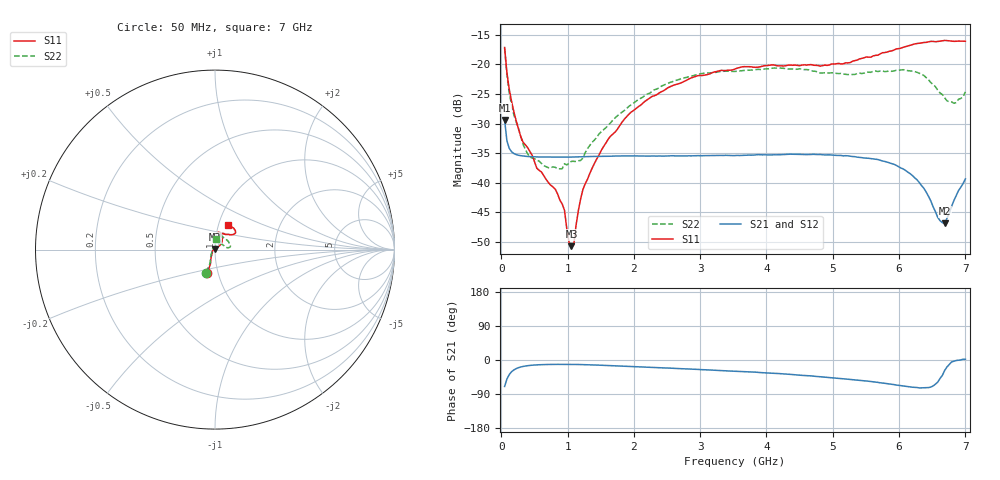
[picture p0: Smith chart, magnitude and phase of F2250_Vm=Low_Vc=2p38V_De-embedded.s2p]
! Integrated Device Technology
! Corporate Headquarters
! 6024 Silver Creek Valley Road
! San Jose, CA 95138  USA
! Phone:  1-408-284-8200
! Toll Free:  1-800-223-1366
! Webpage:  http://www.idt.com/
! Timing and RF Division
! 515 Groton Road, Suite 102
! Westford, MA 01886-6024
! Device:  F2250
! Description: Voltage Variable RF Attenuator
! Frequency:  50.0 -  6000.00 MHz
! Package:  3x3 mm Thin QFN Plastic Package: 16 pin
! Ports:  2 RF, 3 DC
!  Pin  1  = GND
!  Pin  2  = NC
!  Pin  3  = RF1  = Port 1
!  Pin  4  = NC
!  Pin  5  = GND
!  Pin  6  = GND
!  Pin  7  = GND
!  Pin  8  = GND
!  Pin  9  = NC
!  Pin 10  = RF2  = Port 2
!  Pin 11  = NC
!  Pin 12  = GND
!  Pin 13  = GND
!  Pin 14  = VCNTRL
!  Pin 15  = VDD
!  Pin 16  = VMODE
! Vcntrl:  2.380 Volts
! Vmode:  +0.000 Volts
! Vdd:  +3.30  Volts
! Current:  1.177 mA
! Data:  The device was measured on a the F2250 evaluation board which has
!  individual transmission lines to the RF pins.  Data was collected
!  using a calibrated network analyzer.  The evaluation board was
!  de-embedded using a TRL calibration technique.
!  The reference plane is the edge of the package pin.
! Misc:  SN 10
!  Action Tracker AT0258
! Date Measured:  2014-11-26
! Date:  2015-10-15  MJV
! Note:
!  Integrated Device Technology supplies this data as a sample of measured
!  data at the package pin for this product.  Your particular data for this
!  product may vary.
!  Data was taken at 25 degrees C.
!  Integrated Device Technology reserves the right to change this data at anytime.
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# GHz S dB R 50
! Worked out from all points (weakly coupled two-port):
!   201 points, 50 MHz to 7 GHz, reference 50 ohm
!   highest |S21| = -29.41 dB at 50 MHz (marker M1); lowest = -46.9 dB at 6.687 GHz (marker M2)
!   lowest |S11| = -50.7 dB at 1.058 GHz (marker M3), VSWR 1.01, Z = 49.8 + j0.242 ohm
!   |S11| at or under -10 dB: start of sweep to end of sweep
!   |S22| runs from -37.6 to -17.3 dB; largest |S21 - S12| = 6e-05
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0.05  -17.18 -108.6  -29.41 -69.8  -29.41 -69.8  -17.29 -111.0
0.08475  -21.44 -107.5  -32.91 -50.3  -32.91 -50.3  -21.77 -110.1
0.15425  -26.23 -116.6  -34.75 -31.1  -34.75 -31.1  -26.84 -122.2
0.29325  -32.20 -127.8  -35.43 -18.5  -35.42 -18.5  -32.15 -137.2
0.3975  -34.06 -141.8  -35.56 -15.0  -35.55 -15.0  -35.13 -160.3
0.91875  -43.57 158.0  -35.68 -11.5  -35.68 -11.5  -37.62 132.9
0.9535  -44.64 169.7  -35.67 -11.5  -35.68 -11.5  -36.77 130.8
1.023  -50.05 143.8  -35.67 -11.6  -35.67 -11.6  -36.68 115.3
1.05775  -50.68 123.7  -35.66 -11.6  -35.66 -11.6  -36.38 110.1
1.0925  -50.48 89.7  -35.65 -11.7  -35.65 -11.7  -36.37 105.5
1.162  -44.70 57.0  -35.63 -11.9  -35.63 -11.9  -36.28 94.8
1.2315  -41.11 44.2  -35.60 -12.1  -35.60 -12.1  -35.81 85.2
1.6485  -32.12 41.9  -35.51 -14.7  -35.52 -14.7  -29.88 64.2
1.96125  -28.05 42.2  -35.45 -17.2  -35.46 -17.2  -26.82 56.7
2.37825  -24.87 47.3  -35.47 -20.3  -35.47 -20.3  -23.99 56.7
3.525  -20.80 72.5  -35.40 -29.5  -35.40 -29.6  -21.21 74.7
4.7065  -20.16 72.4  -35.19 -42.6  -35.20 -42.6  -21.17 72.2
5.85325  -17.82 40.5  -36.64 -63.3  -36.63 -63.3  -21.14 22.9
6.27025  -16.51 40.1  -39.49 -72.6  -39.49 -72.7  -21.36 9.5
6.68725  -15.99 48.8  -46.85 -27.7  -46.81 -27.5  -25.66 28.4
6.861  -16.13 55.1  -42.18 -1.4  -42.13 -1.3  -26.48 58.0
7  -16.13 63.2  -39.34 1.8  -39.30 1.7  -24.65 83.2
